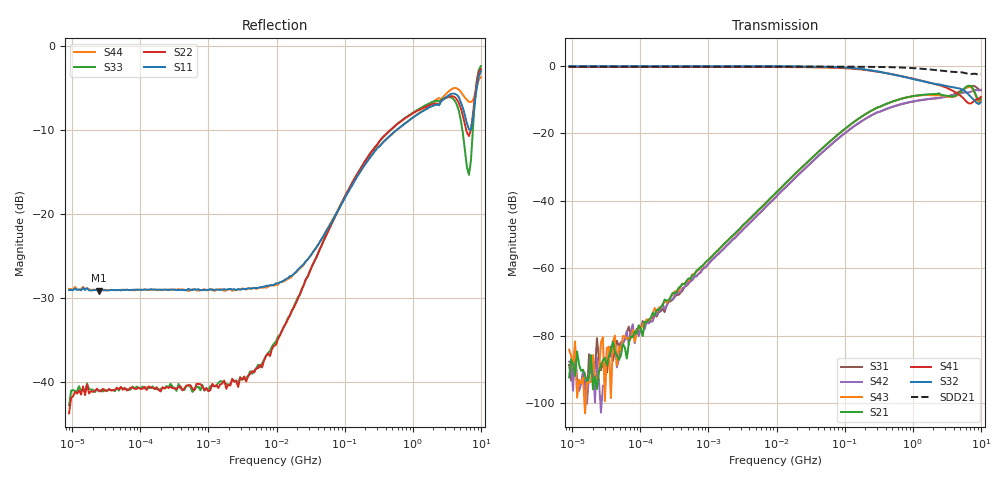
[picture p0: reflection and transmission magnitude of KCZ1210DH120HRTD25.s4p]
! S-Parameter Data Generated by TDK Corporation
! Copyright(C) 2024 TDK Corporation.
! All Rights Reserved.
! TDK P/N: KCZ1210DH120HRTD25 (Signal Line Common Mode Choke/Filter)
! Property: |Zc|=12ohm at 100MHz
! Size(LxWxT): 1.25x1x0.5mm
! Model Type: s2p (Touchstone File Format Version 1.0)
! Frequency: DC=Yes Start=0.009MHz Stop=10000MHz 209points Log-sweep
! Model Generated on May 28, 2024
! Terms and conditions regarding TDK Simulation Models:
! 1)This simulation model is being provided solely for informational
!  purposes. Please refer to the specifications of the products in
!  terms of detailed characteristics of such products.
! 2)In no event shall TDK Corporation of any of its subsidiaries be
!  liable for any loss or damage arising, directly or indirectly,
!  from any information contained in this simulation model, including,
!  but not limited to loss or damages arising from any inaccuracies,
!  omissions or errors in connection with such information.
! 3)Any and all copyrights on this simulation model are owned by
!  TDK Corporation.  Duplication or redistribution of this simulation
!  model without prior written permission from TDK Corporation
!  is prohibited.
! 4)This simulation model is subject to any modification or change
!  without any prior notice.
! 5)Neither TDK Corporation nor any of its subsidiaries shall make any
!  warranty, express or implied, including but not limited to the
!  correctness, implied warranties of merchantability and fitness for
!  a particular purpose with respect to this simulation models.
! 6)The use of this simulation model shall be deemed to have consented
!  to the terms and conditions hereof.
! Port Assignments:
!  1 ---@@@--- 4
!  2 ---@@@--- 3
! Applicable Conditions:
!  Temperature = 25 degC
!  DC Bias Current = 0 A
!  Small Signal Operation
# Hz S MA R 50
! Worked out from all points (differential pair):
!   208 points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, 9 kHz to 10 GHz, reference 50 ohm
!   strongest paths, dB at 9 kHz, 297.2 kHz, 9.811 MHz, 323.9 MHz, 10 GHz:
!     S32: -0.1, -0.1, -0.1, -1.7, -10.7
!     S41: -0.3, -0.3, -0.3, -1.8, -9.1
!     S21: -92.4, -67.3, -37.5, -12.1, -9.8
!     S43: -84.1, -67.8, -37.6, -12.2, -10.2
!     S42: -87.7, -69.3, -38.8, -13.6, -7.0
!     S31: -88.6, -69.3, -38.8, -13.6, -7.2
!   taken as a pair (ports 2,1 in; 3,4 out), SDD21 dB: -0.2, -0.2, -0.2, -0.3, -2.4
!   lowest |S11| = -29.2 dB at 24.68 kHz (marker M1), VSWR 1.07, Z = 53.6 + j0.0158 ohm
!   |S11| at or under -10 dB: start of sweep to 589.3 MHz; 7.04 GHz to 7.149 GHz (109 MHz wide, 1.54 % of centre)
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9000  0.03502 -1.2  3.55e-05 -143.5  1.827e-05 -85.7  0.9649 0.0
      2.411e-05 123.0  0.006471 -24.7  0.9924 0.3  3.132e-05 -123.2
      3.704e-05 -52.2  0.9927 0.3  0.007223 -24.9  1.293e-05 102.9
      0.9644 0.0  4.136e-05 -56.4  6.239e-05 99.7  0.03564 0.8
24679.76  0.03468 0.2  2.017e-05 102.0  4.493e-05 -125.3  0.965 -0.0
          3.046e-05 142.6  0.008817 -2.3  0.9908 0.0  5.604e-05 -106.5
          4.396e-05 -136.4  0.9908 0.0  0.00873 -4.2  1.697e-05 -131.1
          0.9649 -0.0  2.168e-05 -99.4  2.963e-05 175.1  0.03504 0.6
108364  0.03509 0.8  0.000126 89.0  0.0001206 -102.6  0.9647 -0.0
        9.903e-05 84.2  0.009082 -2.5  0.9907 0.0  0.0001231 -65.6
        0.0001655 -90.9  0.9909 0.0  0.009347 -0.3  0.0001518 78.6
        0.9646 -0.0  0.0001442 -86.6  0.0001479 95.4  0.0352 0.4
3577883  0.03559 7.1  0.004825 88.7  0.004194 -91.4  0.9651 -0.4
         0.00481 88.8  0.01 29.7  0.991 -0.3  0.004201 -91.4
         0.004156 -91.0  0.9911 -0.3  0.01057 29.1  0.004764 89.3
         0.9644 -0.3  0.004218 -91.3  0.004804 88.8  0.03526 6.7
2.023111e8  0.1977 41.4  0.1935 53.7  0.165 -132.8  0.8706 -12.7
            0.1932 53.7  0.207 48.8  0.8852 -13.1  0.1656 -132.9
            0.1648 -132.8  0.8852 -13.1  0.2069 48.9  0.1926 53.7
            0.8702 -12.7  0.1659 -132.9  0.1926 53.7  0.1985 41.6
6.679757e9  0.3176 6.1  0.5112 3.7  0.4932 66.4  0.2779 -88.0
            0.5108 3.8  0.2892 -10.4  0.3731 -100.7  0.4067 60.7
            0.4921 66.2  0.3728 -100.7  0.1699 2.0  0.4925 1.8
            0.2785 -88.0  0.4078 60.8  0.4928 1.7  0.4626 7.3
1e10  0.7028 -42.6  0.3232 7.4  0.4354 37.5  0.3491 -150.9
      0.3236 7.5  0.7226 -29.6  0.2915 -153.2  0.4449 41.3
      0.4357 37.6  0.2911 -153.2  0.7541 -21.5  0.3078 18.1
      0.3494 -150.7  0.4447 41.3  0.3077 18.1  0.6482 -20.0
